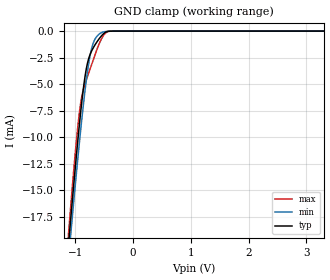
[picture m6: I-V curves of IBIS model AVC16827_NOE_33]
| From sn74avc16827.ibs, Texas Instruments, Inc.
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[Model]   AVC16827_NOE_33
Model_type  Input
Vinl=0.8
Vinh=2.0
| variable   typ   min   max
C_comp   2.51pF   1.72pF   2.93pF
[Temperature Range]   40   100   -40
| Ambient temperature   25   85   -40
[Voltage range]   3.3   3   3.6
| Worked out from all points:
|   GND clamp passes 1 mA (typ) near -0.62 V on its own axis
[GND Clamp]
| AVC16827_NOE_33
|   Voltage   I(typ)   I(min)   I(max)
-3.3V     -175.1mA   -168.3mA   -186.4mA
-1.115V   -19.91mA   -21.27mA   -18.85mA
-1.095V   -18.63mA   -20.05mA   -17.49mA
-1.075V   -17.37mA   -18.85mA   -16.15mA
-990mV    -12.18mA   -13.85mA   -10.78mA
-935mV    -9.059mA   -10.77mA   -7.878mA
-890mV    -6.731mA   -8.379mA   -6.205mA
-820mV    -3.852mA   -5.028mA   -4.756mA
-710mV    -1.78mA    -1.47mA    -3.027mA
-555mV    -494.8uA   -165.2uA   -814uA
-365mV    -4.579uA   -4.897uA   -3.67uA
3.3V      282.5pA    981.5pA    20.95pA
